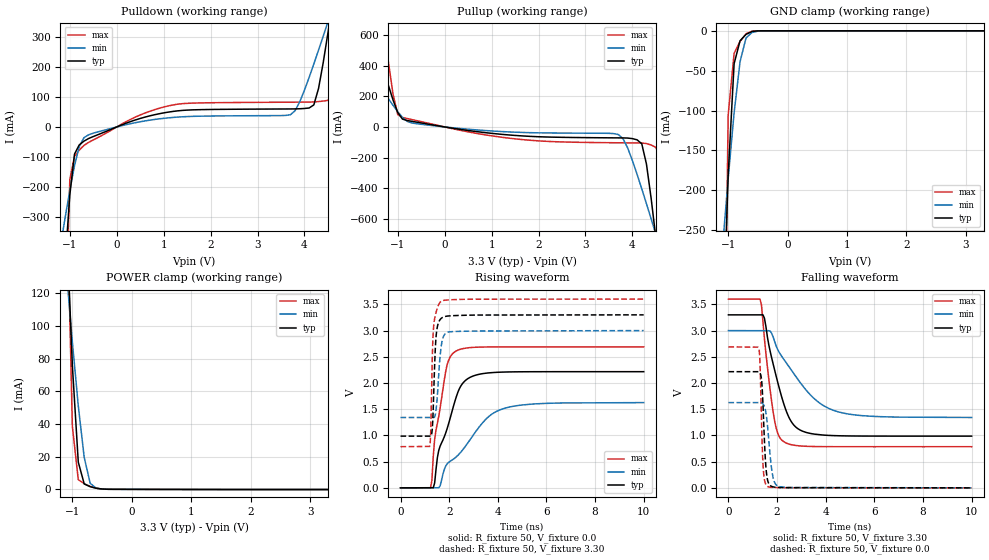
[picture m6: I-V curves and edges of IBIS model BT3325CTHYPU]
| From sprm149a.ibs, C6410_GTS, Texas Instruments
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[Model]   BT3325CTHYPU
Model_type   I/O
Vinh = 2.00
Vinl = 0.80
Enable   Active-Low
Polarity   Non-Inverting
| signals   A, GZ, Y
Vmeas = 1.5
|   typ   min   max
C_comp   1.5797p   1.5046p   1.7659p
|   typ   min   max
[Temperature Range]   25   -40   125
|   typ   min   max
[Voltage Range]   3.30V   3.00V   3.60V
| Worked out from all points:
|   slope of the pulldown table from 0 to 0.495 V, typ, clamps not added: 17.7 ohm
|   slope of the pullup table from 0 to 0.495 V, typ, clamps not added: 21.6 ohm
|   GND clamp passes 1 mA (typ) near -0.60 V on its own axis
|   POWER clamp passes 1 mA (typ) near -0.63 V on its own axis
|   rising waveform, R_fixture 50, V_fixture 0.0: 20-80 % time 838ps typ, 1.71ns min, 494ps max; typ from 0 V to 2.22 V
|   falling waveform, R_fixture 50, V_fixture 3.30: 20-80 % time 773ps typ, 1.6ns min, 430ps max; typ from 3.3 V to 0.987 V
|   rising waveform, R_fixture 50, V_fixture 3.30: 20-80 % time 114ps typ, 164ps min, 98.9ps max; typ from 0.987 V to 3.3 V
|   falling waveform, R_fixture 50, V_fixture 0.0: 20-80 % time 131ps typ, 208ps min, 99.4ps max; typ from 2.22 V to 0 V
[Pulldown]
|   Voltage   I(typ)   I(min)   I(max)
-3.3V     -6.793A    -2.573A    -22.74A
-1.1V     -450.2mA   -301mA     -721mA
-900mV    -90.05mA   -128.3mA   -97.36mA
-600mV    -38.44mA   -26.14mA   -51.28mA
1.2V      51.55mA    31.56mA    73.11mA
3.7V      59.71mA    40.53mA    82.18mA
4.2V      73.24mA    209.2mA    83.11mA
4.5V      311.7mA    348.6mA    88.35mA
4.6V      414.9mA    396.1mA    114.8mA
4.7V      520.9mA    443.9mA    265.2mA
4.8V      628.6mA    491.9mA    481.5mA
6.6V      2.639A     1.373A     5.22A
[GND_clamp]
|   Voltage   I(typ)   I(min)   I(max)
-3.3V     -6.736A    -2.535A    -22.69A
-1.1V     -408.9mA   -276.2mA   -663.1mA
-1V       -181.3mA   -185.5mA   -105.7mA
-900mV    -41.24mA   -103mA     -28.37mA
-800mV    -12.49mA   -38.74mA   -13.33mA
-700mV    -4.472mA   -9.072mA   -3.785mA
-600mV    -854.1uA   -2.124mA   -419.5uA
-400mV    -4.328uA   -46.41uA   -434.3nA
3.3V      177.6pA    2.083uA    133.2pA
[Pullup]
|   Voltage   I(typ)   I(min)   I(max)
-3.3V     2.593A     1.198A     5.964A
-2.2V     1.358A     659.5mA    3.01A
-1.6V     694.9mA    370.7mA    1.424A
-1.3V     373.6mA    230.2mA    661.1mA
-1V       93.86mA    99.05mA    81.11mA
-800mV    41.97mA    36.23mA    54.78mA
3.7V      -71.34mA   -49.45mA   -103.2mA
4.1V      -83.88mA   -308.4mA   -104.2mA
4.5V      -721.2mA   -699.1mA   -132.7mA
4.6V      -990.5mA   -800mA     -203.8mA
4.7V      -1.267A    -901.7mA   -745.3mA
6.6V      -6.788A    -2.882A    -19.69A
[POWER_clamp]
|   Voltage   I(typ)   I(min)   I(max)
-3.3V     2.588A     1.191A     5.962A
-1.1V     164.1mA    133.2mA    197.1mA
-1V       76.16mA    90.45mA    38.61mA
-900mV    16.71mA    51.17mA    5.957mA
-800mV    3.31mA     19.53mA    3.455mA
-700mV    1.625mA    3.736mA    1.82mA
-600mV    707.1uA    738uA      679.1uA
-500mV    198.8uA    185uA      148.9uA
3.3V      -108.4uA   -67.78uA   -162.2uA
[Ramp]
|   I(typ)   I(min)   I(max)
dV/dt_r   1.330/0.839n   0.976/1.712n   1.613/0.493n
dV/dt_f   1.388/0.774n   0.995/1.601n   1.689/0.431n
[Rising Waveform]
R_fixture = 50
V_fixture = 0.0
|  pu_on
|  TIME   V(typ)   V(min)   V(max)
0s        2nV        12nV       1nV
1.234ns   2.499mV    1.683mV    1.411nV
1.29ns    2.499mV    1.837mV    143.4mV
1.403ns   92.15mV    1.837mV    925.2mV
1.572ns   714.1mV    1.837mV    1.367V
1.854ns   1.041V     411.7mV    2.211V
2.305ns   1.753V     596.7mV    2.615V
2.869ns   2.11V      924.4mV    2.675V
4.336ns   2.21V      1.526V     2.689V
10ns      2.216V     1.626V     2.689V
[Falling Waveform]
R_fixture = 50
V_fixture = 3.30
V_fixture_min = 3.00
V_fixture_max = 3.60
|  pd_on
|  TIME   V(typ)   V(min)   V(max)
0s        3.3V       3V         3.6V
1.298ns   3.3V       2.998V     3.6V
1.359ns   3.3V       2.998V     3.489V
1.48ns    3.237V     2.998V     2.848V
1.903ns   2.242V     2.786V     1.27V
2.084ns   1.911V     2.587V     980.2mV
2.326ns   1.532V     2.419V     867.2mV
2.931ns   1.107V     2.022V     800.7mV
4.503ns   994.2mV    1.452V     785.5mV
10ns      986.8mV    1.342V     785.2mV
[Rising Waveform]
R_fixture = 50
V_fixture = 3.30
V_fixture_min = 3.00
V_fixture_max = 3.60
|  pd_off
|  TIME   V(typ)   V(min)   V(max)
0s        986.8mV    1.342V     785.2mV
1.2ns     986.8mV    1.343V     790.5mV
1.241ns   986.8mV    1.343V     1.058V
1.303ns   1.107V     1.343V     2.402V
1.365ns   1.797V     1.343V     3.097V
1.427ns   2.614V     1.387V     3.283V
1.468ns   2.916V     1.514V     3.358V
1.674ns   3.233V     2.702V     3.56V
2.044ns   3.281V     2.978V     3.587V
10ns      3.3V       3V         3.6V
[Falling Waveform]
R_fixture = 50
V_fixture = 0.0
|  pu_off
|  TIME   V(typ)   V(min)   V(max)
0s        2.216V     1.626V     2.689V
1.252ns   2.216V     1.626V     2.654V
1.304ns   2.185V     1.626V     2.286V
1.356ns   2.083V     1.626V     1.352V
1.434ns   1.431V     1.592V     354.3mV
1.525ns   495.2mV    1.473V     77.34mV
1.603ns   162mV      1.198V     28.78mV
1.812ns   22.24mV    253.7mV    8.345mV
2.072ns   7.553mV    27.36mV    4.657mV
10ns      473.7nV    5.393uV    259.4nV
